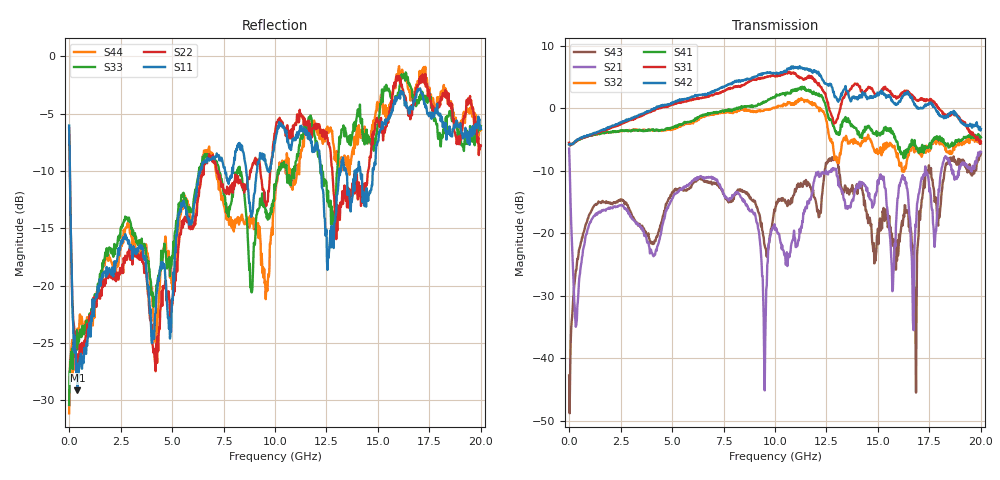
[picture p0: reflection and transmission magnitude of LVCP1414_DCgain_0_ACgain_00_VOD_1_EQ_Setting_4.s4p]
!Agilent Technologies,N5230A,MY46400459,A.07.50.48
!Agilent N5230A: A.07.50.48
!Date: Tuesday, April 17, 2012 18:27:07
!Correction: S11(Full 4 Port(1,2,3,4))
!S12(Full 4 Port(1,2,3,4))
!S13(Full 4 Port(1,2,3,4))
!S14(Full 4 Port(1,2,3,4))
!S21(Full 4 Port(1,2,3,4))
!S22(Full 4 Port(1,2,3,4))
!S23(Full 4 Port(1,2,3,4))
!S24(Full 4 Port(1,2,3,4))
!S31(Full 4 Port(1,2,3,4))
!S32(Full 4 Port(1,2,3,4))
!S33(Full 4 Port(1,2,3,4))
!S34(Full 4 Port(1,2,3,4))
!S41(Full 4 Port(1,2,3,4))
!S42(Full 4 Port(1,2,3,4))
!S43(Full 4 Port(1,2,3,4))
!S44(Full 4 Port(1,2,3,4))
!S4P File: Measurements: <S11,S12,S13,S14>,
!<S21,S22,S23,S24>,
!<S31,S32,S33,S34>,
!<S41,S42,S43,S44>:
# Hz S  dB  R 50
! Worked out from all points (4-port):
!   801 points, 300 kHz to 20 GHz, reference 50 ohm
!   strongest paths, dB at 300 kHz, 5 GHz, 10 GHz, 15 GHz, 20 GHz:
!     S42: -5.8, 0.9, 5.6, 2.4, -3.3
!     S31: -5.5, 0.6, 5.1, 2.1, -5.6
!     S41: -5.6, -3.0, 1.7, -3.9, -4.7
!     S32: -5.8, -3.4, 0.1, -7.3, -5.4
!     S21: -6.5, -14.5, -19.5, -11.5, -7.0
!     S43: -42.8, -13.5, -16.5, -19.3, -7.3
!   lowest |S11| = -29.1 dB at 400.3 MHz (marker M1), VSWR 1.07, Z = 53.2 + j1.56 ohm
!   |S11| at or under -10 dB: 37.44 MHz to 6.373 GHz (6.336 GHz wide, 198 % of centre); 12.22 GHz to 13.12 GHz (895.2 MHz wide, 7.07 % of centre); 14.14 GHz to 14.75 GHz (602.8 MHz wide, 4.17 % of centre)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
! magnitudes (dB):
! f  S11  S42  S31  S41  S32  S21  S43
! 300 kHz  -6.0  -5.8  -5.5  -5.6  -5.8  -6.5  -42.8
! 400.3 MHz  -29.1  -5.0  -5.0  -5.1  -5.1  -31.7  -24.1
! 9.95 GHz  -8.1  5.6  5.2  1.8  0.1  -19.1  -16.6
! 12.85 GHz  -16.7  2.6  -2.3  -2.8  -7.0  -9.6  -7.9
! 16.8 GHz  -3.6  0.7  1.6  -5.8  -6.4  -20.2  -28.9
! 17.4 GHz  -5.0  0.7  1.3  -6.3  -6.5  -10.4  -10.0
! 20 GHz  -6.3  -3.3  -5.6  -4.7  -5.4  -7.0  -7.3
